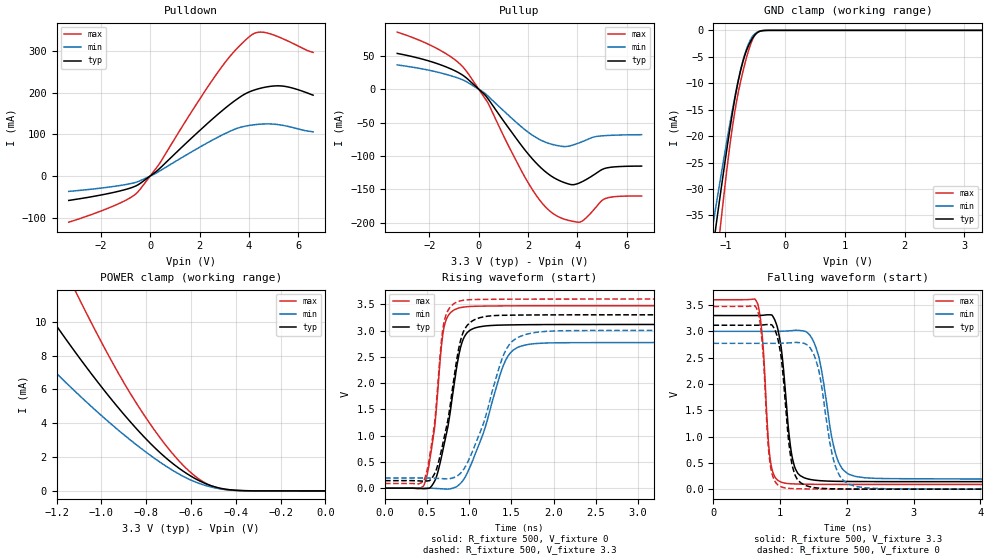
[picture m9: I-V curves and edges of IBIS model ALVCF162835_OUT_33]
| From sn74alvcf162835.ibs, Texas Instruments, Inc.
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[Model]   ALVCF162835_OUT_33
Model_type  3-state
Enable   Active-Low
Vref =   0
Rref =   500
Cref =   50p
Vmeas =   1.5
| variable   typ   min   max
C_comp   2.89pF   2.62pF   3.31pF
| C_pullup   3.14pF   2.30pF   4.21pF
| C_pulldown   2.22pF   1.91pF   2.89pF
| C_tri-state   2.89pF   2.62pF   3.31pF
[Temperature Range]   40   100   -40
| Ambient temperature   25   85   -40
[Voltage range]   3.3   3   3.6
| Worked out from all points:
|   slope of the pulldown table from 0 to 0.495 V, typ, clamps not added: 20.2 ohm
|   slope of the pullup table from 0 to 0.495 V, typ, clamps not added: 24.1 ohm
|   GND clamp passes 1 mA (typ) near -0.52 V on its own axis
|   POWER clamp passes 1 mA (typ) near -0.62 V on its own axis
|   rising waveform, R_fixture 500, V_fixture 0: 20-80 % time 198ps typ, 330ps min, 128ps max; typ from 0 V to 3.12 V
|   falling waveform, R_fixture 500, V_fixture 3.3: 20-80 % time 142ps typ, 222ps min, 99.2ps max; typ from 3.3 V to 0.143 V
|   rising waveform, R_fixture 500, V_fixture 3.3: 20-80 % time 200ps typ, 332ps min, 128ps max; typ from 0.143 V to 3.3 V
|   falling waveform, R_fixture 500, V_fixture 0: 20-80 % time 140ps typ, 216ps min, 99.2ps max; typ from 3.12 V to 0 V
[GND Clamp]
| ALVCF162835_OUT_33
|   Voltage   I(typ)   I(min)   I(max)
-3.3V     -231.3mA   -196.9mA   -290mA
-1.21V    -41.31mA   -36.83mA   -50.32mA
-1.155V   -36.76mA   -32.99mA   -44.48mA
-1.1V     -32.26mA   -29.21mA   -38.74mA
-1.075V   -30.25mA   -27.51mA   -36.17mA
-965mV    -21.64mA   -20.2mA    -25.32mA
-890mV    -16.15mA   -15.46mA   -18.84mA
-760mV    -8.298mA   -8.123mA   -10.4mA
-605mV    -2.692mA   -2.342mA   -3.539mA
-525mV    -1.132mA   -849.3uA   -1.245mA
-455mV    -359.4uA   -272.2uA   -291.3uA
3.3V      1.433nA    4.434uA    123.8pA
[POWER Clamp]
| ALVCF162835_OUT_33
|   Voltage   I(typ)   I(min)   I(max)
-3.3V     60.8mA     42.78mA    83.8mA
-1.54V    16.66mA    11.72mA    24.13mA
-1.51V    16.02mA    11.28mA    23.21mA
-1.3V     11.7mA     8.29mA     16.96mA
-1.115V   8.181mA    5.861mA    11.8mA
-1.09V    7.73mA     5.549mA    11.13mA
-935mV    5.092mA    3.717mA    7.225mA
-800mV    3.067mA    2.288mA    4.308mA
-680mV    1.608mA    1.204mA    2.176mA
-580mV    721uA      528.1uA    857.4uA
-445mV    102uA      83.45uA    72.96uA
-48.03fV  1.433nA    2.89nA     157.5pA
[Pulldown]
| ALVCF162835_OUT_33
|   Voltage   I(typ)   I(min)   I(max)
-3.3V     -58.79mA   -37.03mA   -111.2mA
-1.415V   -38.61mA   -24.57mA   -70.31mA
-850mV    -29.86mA   -18.99mA   -53.84mA
-515mV    -21.87mA   -13.9mA    -39.24mA
370mV     17.44mA    11.63mA    29.32mA
1.71V     93.35mA    59.35mA    158mA
2.82V     152.6mA    95.88mA    256.5mA
3.42V     181.1mA    112.6mA    301.1mA
4.1V      204.7mA    122.6mA    339.5mA
4.55V     212.6mA    125.2mA    346.5mA
5.285V    217mA      123mA      333mA
6.6V      194.7mA    106.4mA    297.9mA
[Pullup]
| ALVCF162835_OUT_33
|   Voltage   I(typ)   I(min)   I(max)
-3.3V     53.58mA    36.36mA    85.57mA
-1.65V    37.9mA     25.36mA    60.13mA
-585mV    19.32mA    12.86mA    31.03mA
370mV     -13.99mA   -10.16mA   -20.38mA
1.23V     -59.06mA   -39.9mA    -86.58mA
2.09V     -100.9mA   -66.78mA   -145.6mA
2.59V     -120.2mA   -77.69mA   -171.7mA
3.05V     -132.8mA   -83.45mA   -187.4mA
3.725V    -143mA     -84.73mA   -197.4mA
4.095V    -140.4mA   -80.16mA   -199.3mA
5.115V    -118.8mA   -69.67mA   -164.3mA
6.6V      -115.3mA   -68.25mA   -160.3mA
[Ramp]
| ALVCF162835_OUT_33
| variable   typ   min   max
dV/dt_r   1.88/2.00E-10   1.67/3.35E-10   2.09/1.29E-10
dV/dt_f   1.90/1.43E-10   1.70/2.28E-10   2.11/1.04E-10
R_load = 500
[Rising Waveform]
| ALVCF162835_OUT_33
R_fixture =   500
C_fixture =   0
L_fixture =   0
V_fixture =   0
V_fixture_min = 0
V_fixture_max = 0
|   Time   V(typ)   V(min)   V(max)
0s        3.443uV    -7.417uV   5.242uV
455ps     -9.946mV   488.1uV    39.58mV
585ps     122.7mV    -3.556mV   1.11V
665ps     558.7mV    -11.04mV   2.628V
705ps     858.9mV    -14.87mV   3.095V
875ps     2.523V     59.58mV    3.429V
960ps     2.929V     238.3mV    3.453V
1.44ns    3.107V     2.46V      3.47V
1.79ns    3.113V     2.753V     3.472V
24.99ns   3.116V     2.772V     3.473V
[Falling Waveform]
| ALVCF162835_OUT_33
R_fixture =   500
C_fixture =   0
L_fixture =   0
V_fixture =   3.3
V_fixture_min = 3
V_fixture_max = 3.6
|   Time   V(typ)   V(min)   V(max)
0s        3.3V       3V         3.6V
660ps     3.301V     3V         3.531V
860ps     3.313V     2.999V     485.8mV
1.005ns   2.771V     3.001V     139.6mV
1.11ns    1.348V     3.007V     107.4mV
1.3ns     257mV      3.016V     96.31mV
1.57ns    164.3mV    2.557V     91.82mV
1.875ns   148.4mV    513.3mV    90.2mV
2.27ns    144.2mV    216mV      89.62mV
24.99ns   143.2mV    193.6mV    89.5mV
[Rising Waveform]
| ALVCF162835_OUT_33
R_fixture =   500
C_fixture =   0
L_fixture =   0
V_fixture =   3.3
V_fixture_min = 3
V_fixture_max = 3.6
|   Time   V(typ)   V(min)   V(max)
0s        143.2mV    193.5mV    89.51mV
455ps     133.3mV    193.9mV    129.5mV
585ps     266.6mV    189.9mV    1.199V
665ps     693.1mV    182.6mV    2.732V
705ps     986.2mV    179.1mV    3.193V
875ps     2.659V     254.7mV    3.557V
960ps     3.064V     429.7mV    3.583V
1.45ns    3.292V     2.673V     3.598V
1.91ns    3.299V     2.986V     3.599V
24.99ns   3.3V       3V         3.6V
[Falling Waveform]
| ALVCF162835_OUT_33
R_fixture =   500
C_fixture =   0
L_fixture =   0
V_fixture =   0
V_fixture_min = 0
V_fixture_max = 0
|   Time   V(typ)   V(min)   V(max)
0s        3.116V     2.772V     3.473V
660ps     3.116V     2.772V     3.402V
855ps     3.126V     2.771V     432.9mV
1.005ns   2.589V     2.773V     50.55mV
1.11ns    1.138V     2.778V     17.17mV
1.305ns   122.7mV    2.782V     6.47mV
1.555ns   22.78mV    2.37V      2.411mV
1.855ns   5.233mV    345mV      750.3uV
2.275ns   1.007mV    25.73mV    123.7uV
24.99ns   9.55uV     13.08uV    3.982uV
